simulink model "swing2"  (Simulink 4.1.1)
settings: Solver=ode45  StartTime=0.0  StopTime=10.0  MaxStep=0.01  RelTol=1e-3
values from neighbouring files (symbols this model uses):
  f = input('Frequency [default = 1.0] =')    [Actac.m]    (also in alternator.m = getframe(gcf); brushlessdcB.m = getframe(gca); brushlessdcnew.m = getframe(gca); calc0.m = f+dfa*ti/6)
  H = 0.60    (= 0.6)    [IMabc2.m]    (also in IMcur0.m = 0.3; imdef0vec.m = 0.3; imdef1vec.m = 0.3; imdef2vec.m = 0.3)
  V = [Vas 0 0].'    [Actac.m]    (also in acttrcalc1.m = str2num(get(h,'string')); im3d.m = eval(get(hVs,'String')); IMabc2.m = [vas vbs vcs 0 0 0]'; IMabcf0.m = [vas vbs vcs 0 0 0]')
undefined symbols (not defined in the file or in its folder): Pm, Tc, Xafter, Xduring

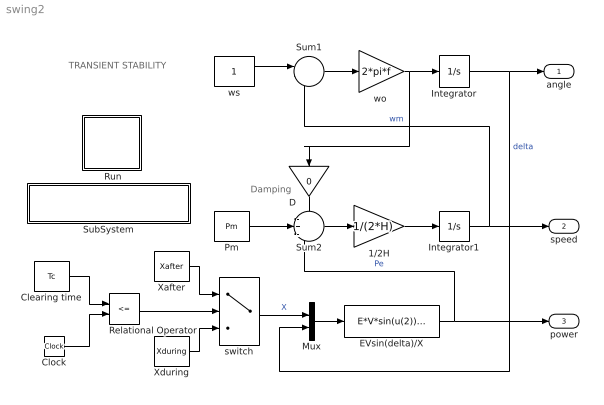
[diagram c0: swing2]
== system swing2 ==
  note: TRANSIENT STABILITY
  note: Damping
  " Run" : Subsystem
  1/2H : Gain  Gain=1/(2*H)  Multiplication=Element-wise(K.*u)  SaturateOnIntegerOverflow=on
  Clearing time : Constant  Value=Tc
  Clock : Clock
  D : Gain  Orientation=down  Gain=0  Multiplication=Element-wise(K.*u)  SaturateOnIntegerOverflow=on
  EVsin(delta)/X : Fcn  Expr=E*V*sin(u(2))/u(1)
  Integrator : Integrator  ExternalReset=none  InitialConditionSource=internal  InitialCondition=0  LimitOutput=off  UpperSaturationLimit=inf  LowerSaturationLimit=-inf  ShowSaturationPort=off  ShowStatePort=off  AbsoluteTolerance=auto
  Integrator1 : Integrator  ExternalReset=none  InitialConditionSource=internal  InitialCondition=0  LimitOutput=off  UpperSaturationLimit=inf  LowerSaturationLimit=-inf  ShowSaturationPort=off  ShowStatePort=off  AbsoluteTolerance=auto
  Mux : Mux  Inputs=2
  Pm : Constant  Value=Pm
  Relational Operator : RelationalOperator  Operator=<=
  SubSystem : Subsystem
  Sum1 : Sum  Inputs=|-+  SaturateOnIntegerOverflow=on
  Sum2 : Sum  Inputs=-+-  SaturateOnIntegerOverflow=on
  Xafter : Constant  Value=Xafter
  Xduring : Constant  Value=Xduring
  switch : Switch  Threshold=0.5
  "wo " : Gain  Gain=2*pi*f  Multiplication=Element-wise(K.*u)  SaturateOnIntegerOverflow=on
  ws : Constant  Value=1
  angle : Outport  Port=1
  speed : Outport  Port=2
  power : Outport  Port=3
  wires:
  ws/1 -> Sum1/1
  Integrator/1 -> Mux/2, angle/1  "delta"
  Sum1/1 -> "wo "/1
  Clearing time/1 -> Relational Operator/1
  Xafter/1 -> switch/1
  Xduring/1 -> switch/3
  Relational Operator/1 -> switch/2
  switch/1 -> Mux/1  "X"
  Clock/1 -> Relational Operator/2
  Mux/1 -> EVsin(delta)/X/1
  Sum2/1 -> 1/2H/1
  1/2H/1 -> Integrator1/1
  Integrator1/1 -> Sum1/2, speed/1  "wm"
  Pm/1 -> Sum2/2
  D/1 -> Sum2/1
  "wo "/1 -> Integrator/1, D/1
  EVsin(delta)/X/1 -> power/1, Sum2/3  "Pe"

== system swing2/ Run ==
  note: Double click the block to enter the parameters and initial conditions and run the simulation
  note: This demo simulates the transient stability problem in a single machine connected to an infinite bus. A sudden disturbance occurs which modifies the electrical output Pe while the mechanical input Pm remains constant. Swings curves are generated for specified clearing times Tc. Power-angle curves are also exhibited.

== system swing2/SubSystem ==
